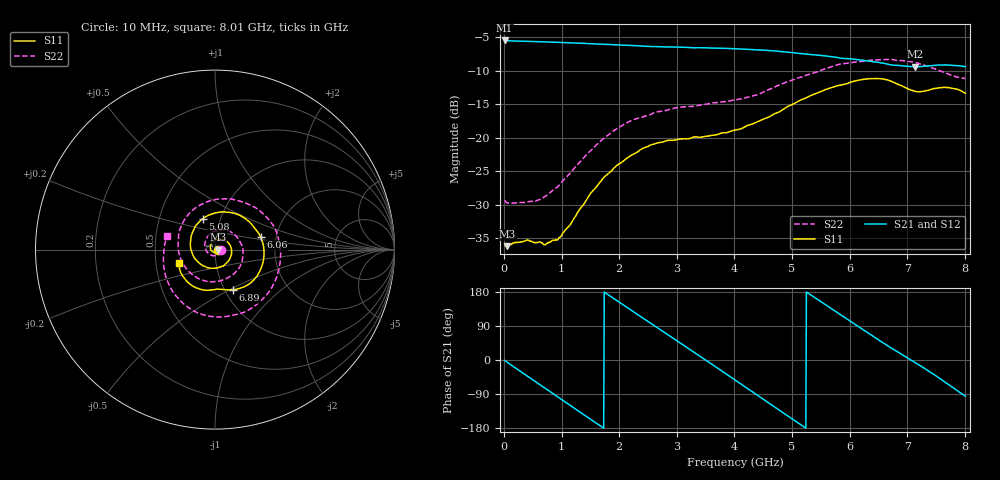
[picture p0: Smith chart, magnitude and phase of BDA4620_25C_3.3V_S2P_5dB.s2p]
!Agilent Technologies,E5071B,MY42404982,A.09.10
!Date: Wed May 06 08:57:02 2026
!Data & Calibration Information:
!Freq	S11:SOLT2(ON)	S21:SOLT2(ON)	S12:SOLT2(ON)	S22:SOLT2(ON)
# Hz S RI R 50
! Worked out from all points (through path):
!   801 points, 10 MHz to 8.01 GHz, reference 50 ohm
!   highest |S21| = -5.45 dB at 10 MHz (marker M1); lowest = -9.4 dB at 7.14 GHz (marker M2)
!   group delay of S21, straight-line fit = 283 ps
!   lowest |S11| = -36.2 dB at 60 MHz (marker M3), VSWR 1.03, Z = 51.6 - j0.129 ohm
!   |S11| at or under -10 dB: start of sweep to end of sweep
!   |S22| runs from -29.8 to -8.3 dB; largest |S21 - S12| = 0.0024
!   S11 on the Smith chart (normalised r, x): 10 MHz: 1.03, -0.00; 5.08 GHz: 0.82, +0.29; 6.06 GHz: 1.66, +0.25; 6.89 GHz: 1.10, -0.52; 8.01 GHz: 0.66, -0.10
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1e7  0.0161 -0.000963  0.5338 -0.0115  0.5346 -0.0117  0.034 -0.00267
6e7  0.0154 -0.00125  0.5284 -0.0607  0.5296 -0.0618  0.0321 -0.00566
3.6e8  0.0141 -0.0093  0.4151 -0.3237  0.4152 -0.3245  0.0197 -0.0263
7.3e8  0.000146 -0.0161  0.1211 -0.5062  0.121 -0.5068  -0.0164 -0.0331
1.03e9  -0.0176 -0.00846  -0.156 -0.4906  -0.1567 -0.4909  -0.0474 -0.00902
1.35e9  -0.0263 0.0157  -0.394 -0.3214  -0.3941 -0.322  -0.0549 0.0405
1.65e9  -0.014 0.0433  -0.4962 -0.0732  -0.497 -0.0734  -0.0257 0.0885
1.94e9  0.0157 0.059  -0.4615 0.1801  -0.4624 0.1807  0.0332 0.1107
2.32e9  0.063 0.0468  -0.2412 0.423  -0.2422 0.4232  0.1174 0.0764
2.68e9  0.0919 0.00146  0.0552 0.4765  0.0556 0.477  0.1565 -0.00672
3e9  0.0827 -0.0499  0.3002 0.3699  0.3008 0.3699  0.139 -0.0948
3.39e9  0.0353 -0.0947  0.4623 0.0919  0.4628 0.0911  0.0443 -0.1691
4.01e9  -0.0785 -0.0825  0.2806 -0.368  0.2805 -0.3687  -0.1605 -0.1053
4.51e9  -0.1371 0.0186  -0.1126 -0.4377  -0.1136 -0.438  -0.2011 0.0922
5.08e9  -0.0691 0.1711  -0.4116 -0.1228  -0.4123 -0.1225  -0.00717 0.2777
5.35e9  0.0201 0.2081  -0.4104 0.0782  -0.4107 0.0789  0.1328 0.2715
6.06e9  0.2539 0.0713  -0.0507 0.384  -0.0501 0.3849  0.366 -0.0244
6.68e9  0.1833 -0.1964  0.2871 0.2059  0.2885 0.2057  0.1881 -0.3362
6.89e9  0.1014 -0.2242  0.3323 0.0962  0.3336 0.0956  0.0632 -0.3729
7.14e9  0.0285 -0.2205  0.3366 -0.0421  0.3373 -0.0434  -0.0962 -0.3525
7.57e9  -0.0972 -0.2155  0.2277 -0.2658  0.2281 -0.2667  -0.2682 -0.1672
8.01e9  -0.2014 -0.0754  -0.033 -0.3383  -0.0339 -0.3395  -0.2661 0.0764
